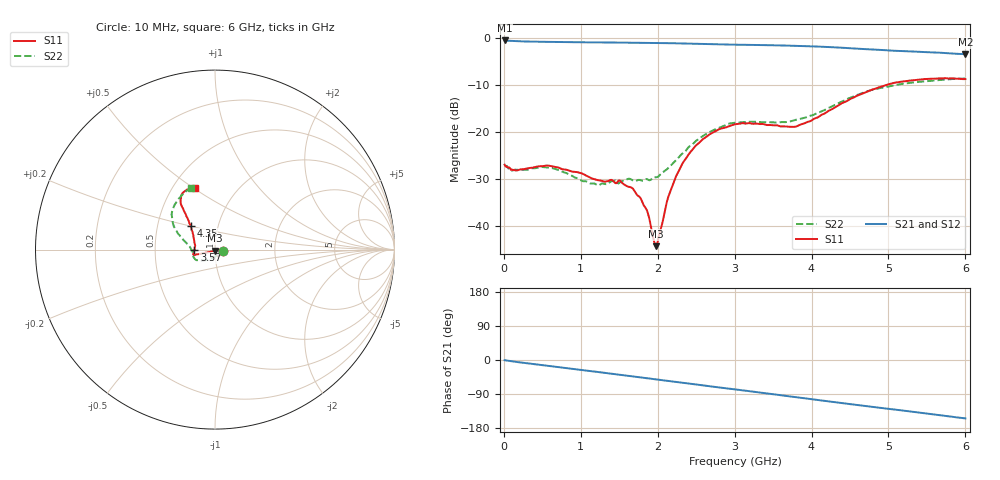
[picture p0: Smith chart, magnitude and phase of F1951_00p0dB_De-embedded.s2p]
! Integrated Device Technology
! Corporate Headquarters
! 6024 Silver Creek Valley Road
! San Jose, CA 95138  USA
! Phone:  1-408-284-8200
! Toll Free:  1-800-223-1366
! Webpage:  http://www.idt.com/
! Timing and RF Division
! 515 Groton Road, Suite 102
! Westford, MA 01886-6024
! Device:  F1951
! Description: 6-bit 0.5 dB Digital Step Attenuator
! Frequency:  100.0 -  4000.00 MHz
! Package:  4x4 mm Thin QFN Plastic Package: 24 pin
! Ports:  2 RF, 6 DC
!  Pin  1  = NC
!  Pin  2  = RF1  =  Port 1
!  Pin  3  = GND
!  Pin  4  = NC
!  Pin  5  = Serial Data Out (SDO)
!  Pin  6  = NC
!  Pin  7  = Reset Bar ( RSTb)
!  Pin  8  = Clock (CLK)
!  Pin  9  = Chip Select Bar (CSb)
!  Pin 10  = NC
!  Pin 11  = Serial Data In (SDI)
!  Pin 12  = NC
!  Pin 13  = NC
!  Pin 14  = VDD
!  Pin 15  = NC
!  Pin 16  = GND
!  Pin 17  = RF2  =  Port 2
!  Pin 18  = NC
!  Pin 19  = GND
!  Pin 20  = GND
!  Pin 21  = GND
!  Pin 22  = GND
!  Pin 23  = GND
!  Pin 24  = GND
! State:  0
! Atten State:  0.0 dB
! Voltage:  +3.30 Volts
! Current:  0.474 mA
! Data:  The device was measured on a F195X evaluation board which has
!  individual transmission lines to the RF pins.  Data was collected
!  de-embedded using a Automatic Fixture Removal [AFR] (Keysight Technologies).
!  The reference plane is the edge of the package pin.
! Misc:  Lot Code  1225BCA
!  Action Tracker AT0399
! Date Measured:  2018-09-13
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# GHz S dB R 50
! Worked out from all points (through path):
!   600 points, 10 MHz to 6 GHz, reference 50 ohm
!   highest |S21| = -0.61 dB at 10 MHz (marker M1); lowest = -3.5 dB at 6 GHz (marker M2)
!   group delay of S21, straight-line fit = 71.3 ps
!   lowest |S11| = -44.4 dB at 1.98 GHz (marker M3), VSWR 1.01, Z = 50.2 - j0.581 ohm
!   |S11| at or under -10 dB: start of sweep to 4.992 GHz
!   |S22| runs from -31.5 to -8.7 dB; largest |S21 - S12| = 0.001
!   S11 on the Smith chart (normalised r, x): 10 MHz: 1.09, -0.01; 3.57 GHz: 0.79, -0.00; 4.35 GHz: 0.74, +0.20; 6 GHz: 0.64, +0.51
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0.01  -27.06 -7.0  -0.61 -0.5  -0.61 -0.5  -27.12 -8.4
0.16  -28.29 -40.4  -0.77 -5.0  -0.77 -5.0  -28.12 -42.5
0.64  -27.43 -64.9  -0.93 -17.1  -0.93 -17.1  -27.81 -70.1
1.01  -28.88 -46.2  -1.00 -26.4  -1.00 -26.4  -30.45 -54.6
1.23  -30.36 -28.9  -1.03 -31.8  -1.03 -31.8  -31.46 -33.7
1.51  -30.47 -6.6  -1.07 -38.8  -1.08 -38.8  -30.82 -18.6
1.67  -32.04 -4.9  -1.09 -43.0  -1.09 -43.0  -30.35 -24.4
1.85  -36.45 -16.9  -1.12 -47.6  -1.13 -47.6  -30.11 -45.2
1.95  -43.19 -48.1  -1.14 -50.2  -1.15 -50.2  -29.71 -62.7
1.98  -44.40 -73.7  -1.15 -51.0  -1.15 -51.0  -29.74 -66.9
2.01  -42.60 -105.8  -1.16 -51.8  -1.16 -51.8  -29.55 -73.1
2.15  -33.36 -148.9  -1.19 -55.4  -1.19 -55.4  -27.57 -96.6
2.25  -29.16 -155.5  -1.22 -58.1  -1.22 -58.1  -25.91 -110.4
2.36  -25.91 -160.1  -1.26 -61.0  -1.26 -61.0  -24.22 -121.2
2.66  -20.77 -164.3  -1.36 -68.8  -1.37 -68.8  -20.22 -141.1
3.01  -18.43 -165.9  -1.50 -77.7  -1.50 -77.6  -18.12 -155.9
3.57  -18.77 -179.1  -1.66 -92.0  -1.67 -92.1  -18.10 -173.7
3.78  -19.00 168.9  -1.77 -97.6  -1.77 -97.5  -17.58 179.5
4.01  -17.53 152.0  -1.87 -103.6  -1.87 -103.6  -16.53 170.9
4.35  -14.44 136.0  -2.12 -112.5  -2.12 -112.5  -13.95 160.2
5.01  -9.92 126.7  -2.76 -129.1  -2.76 -129.1  -10.41 142.5
6  -8.84 108.1  -3.53 -154.1  -3.53 -154.1  -8.69 111.4
